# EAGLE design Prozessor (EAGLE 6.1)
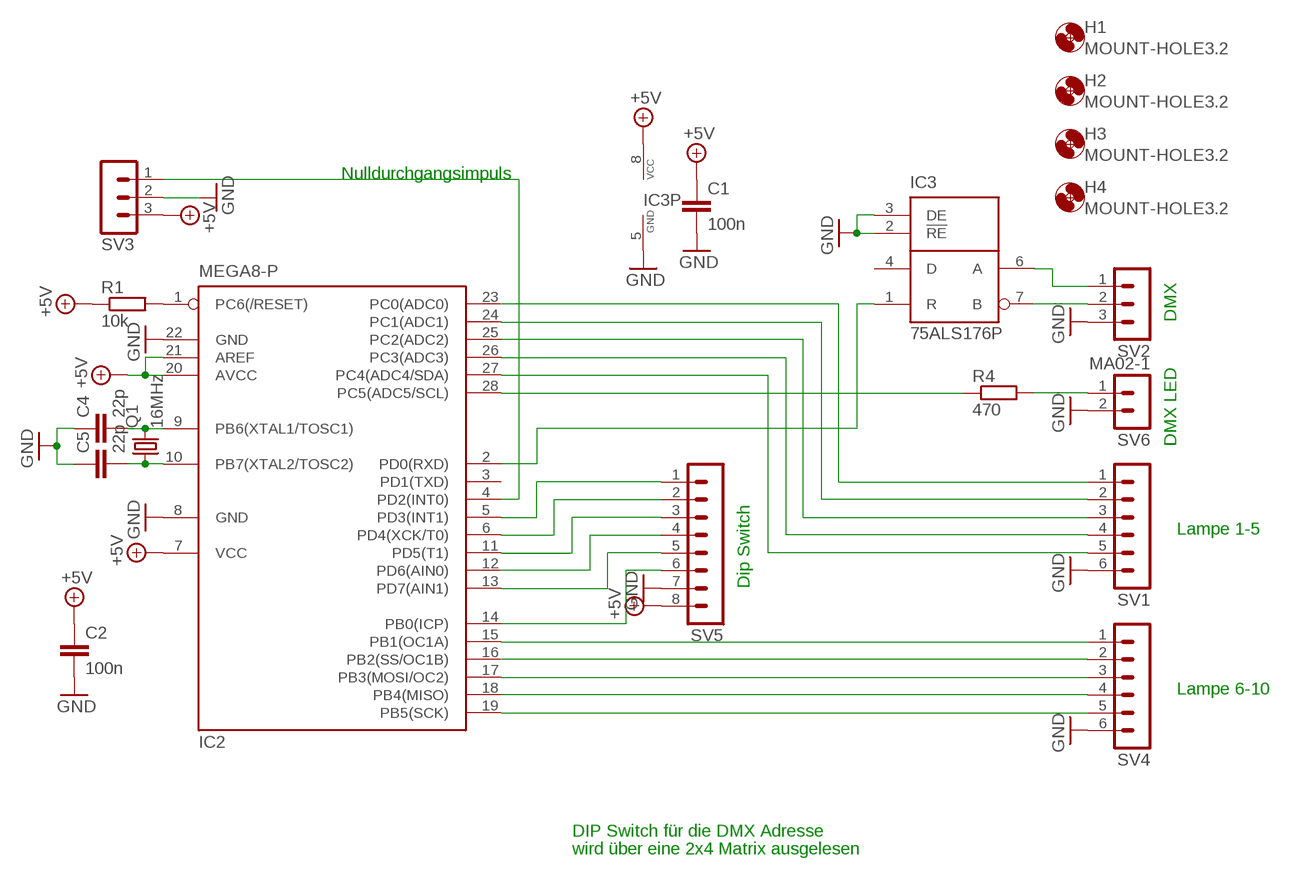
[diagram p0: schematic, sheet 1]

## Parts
C1  100n  C-EU050-025X075  [C050-025X075]
C2  100n  C-EU050-025X075  [C050-025X075]
C4  22p  C-EU025-025X050  [C025-025X050]
C5  22p  C-EU025-025X050  [C025-025X050]
H1  MOUNT-HOLE3.2  [3,2]
H2  MOUNT-HOLE3.2  [3,2]
H3  MOUNT-HOLE3.2  [3,2]
H4  MOUNT-HOLE3.2  [3,2]
IC2  MEGA8-P  [DIL28-3]
IC3  75ALS176P  [DIL08]
Q1  16MHz  CRYSTALHC49U70  [HC49U70]
R1  10k  R-EU_0204/7  [0204/7]
R4  470  R-EU_0204/7  [0204/7]
SV1  MA06-1  [MA06-1]
SV2  MA03-1  [MA03-1]
SV3  MA03-1  [MA03-1]
SV4  MA06-1  [MA06-1]
SV5  MA08-1  [MA08-1]
SV6  MA02-1  [MA02-1]

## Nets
+5V: C1.1 C2.1 IC2.7(VCC) IC2.20(AVCC) IC2.21(AREF) IC3.8(VCC) R1.1 SV3.3 SV5.8
GND: C1.2 C2.2 C4.1 C5.1 IC2.8(GND) IC2.22(GND) IC3.2(!RE) IC3.3(DE) IC3.5(GND) SV1.6 SV2.3 SV3.2 SV4.6 SV5.7 SV6.2
N$1: IC2.12(PD6(AIN0)) SV5.4
N$2: IC2.13(PD7(AIN1)) SV5.5
N$3: IC2.11(PD5(T1)) SV5.3
N$4: IC2.6(PD4(XCK/T0)) SV5.2
N$5: IC2.5(PD3(INT1)) SV5.1
N$6: IC2.27(PC4(ADC4/SDA)) SV1.5
N$7: IC2.23(PC0(ADC0)) SV1.1
N$8: IC2.4(PD2(INT0)) SV3.1
N$9: R4.2 SV6.1
N$10: C4.2 IC2.9(PB6(XTAL1/TOSC1)) Q1.2
N$11: C5.2 IC2.10(PB7(XTAL2/TOSC2)) Q1.1
N$12: IC2.14(PB0(ICP)) SV5.6
N$13: IC2.19(PB5(SCK)) SV4.5
N$14: IC2.18(PB4(MISO)) SV4.4
N$15: IC2.17(PB3(MOSI/OC2)) SV4.3
N$16: IC2.16(PB2(SS/OC1B)) SV4.2
N$17: IC2.15(PB1(OC1A)) SV4.1
N$18: IC2.1(PC6(/RESET)) R1.2
N$19: IC2.24(PC1(ADC1)) SV1.2
N$20: IC2.25(PC2(ADC2)) SV1.3
N$21: IC2.26(PC3(ADC3)) SV1.4
N$23: IC2.2(PD0(RXD)) IC3.1(R)
N$24: IC3.6(A) SV2.1
N$25: IC3.7(B) SV2.2
N$27: IC2.28(PC5(ADC5/SCL)) R4.1
Unconnected: IC2.3(PD1(TXD)) IC3.4(D)

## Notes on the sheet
- Nulldurchgangsimpuls
- DMX
- DMX LED
- Lampe 1-5
- Dip Switch
- Lampe 6-10
- DIP Switch für die DMX Adresse
- wird über eine 2x4 Matrix ausgelesen

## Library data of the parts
C1 C2 = rcl:C-EU: CAPACITOR, European symbol
C4 C5 = resistor:C-EU: CAPACITOR, European symbol
H1-H4 = holes:MOUNT-HOLE: MOUNTING HOLE with drill center marker
IC2 = atmel:MEGA8-P: MICROCONTROLLER 8 Kbytes FLASH, 1 kbytes SRAM, 512 bytes EEPROM, USART, 4-channel 10 bit ADC, 2-channel 8 bit ADC Pin compatible with Atmega48, ATMega88, ATMega168 Source: avr.lbr
IC3 = texas:75ALS176: DIFFERENTIAL BUS TRANSCEIVERS TIA/EIA-422-B, TIA/EIA-422-B + TIA/EIA-422-B TIA/EIA-422-B Operate at Data Rates up to 35 Mbaud Source: http://focus.ti.com/lit/ds/symlink/sn65als176.pdf
Q1 = crystal:CRYSTAL: CRYSTAL
R1 R4 = resistor:R-EU_: RESISTOR, European symbol
SV1 SV4 = con-lstb:MA06-1: PIN HEADER; OC_FARNELL: unknown; OC_NEWARK: unknown
SV2 SV3 = con-lstb:MA03-1: PIN HEADER; OC_FARNELL: unknown; OC_NEWARK: unknown
SV5 = con-lstb:MA08-1: PIN HEADER; OC_FARNELL: unknown; OC_NEWARK: unknown
SV6 = con-lstb:MA02-1: PIN HEADER

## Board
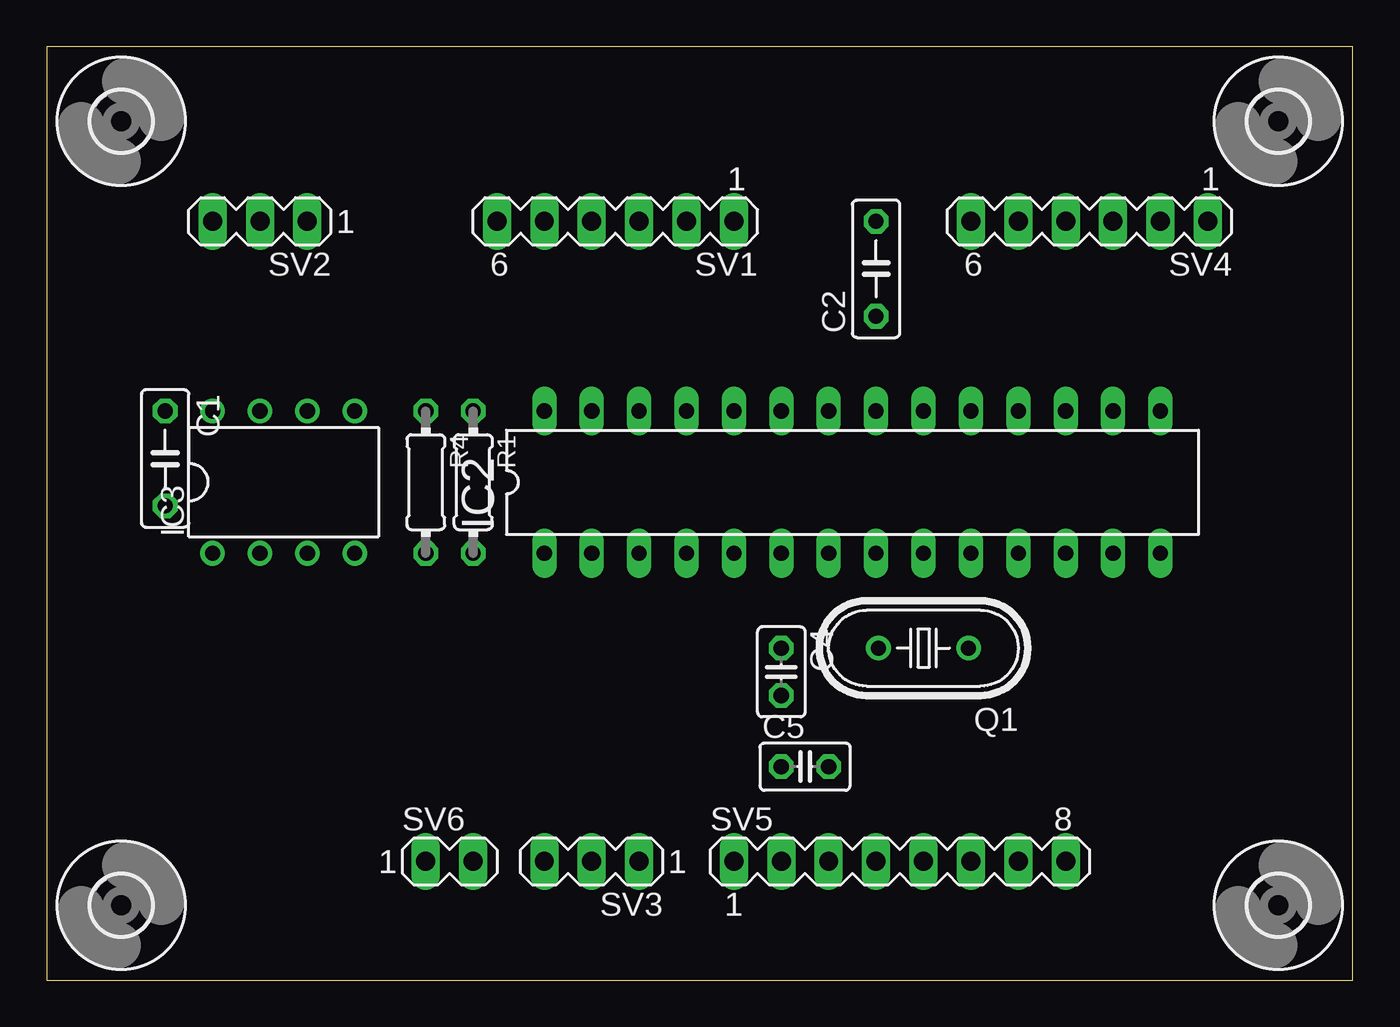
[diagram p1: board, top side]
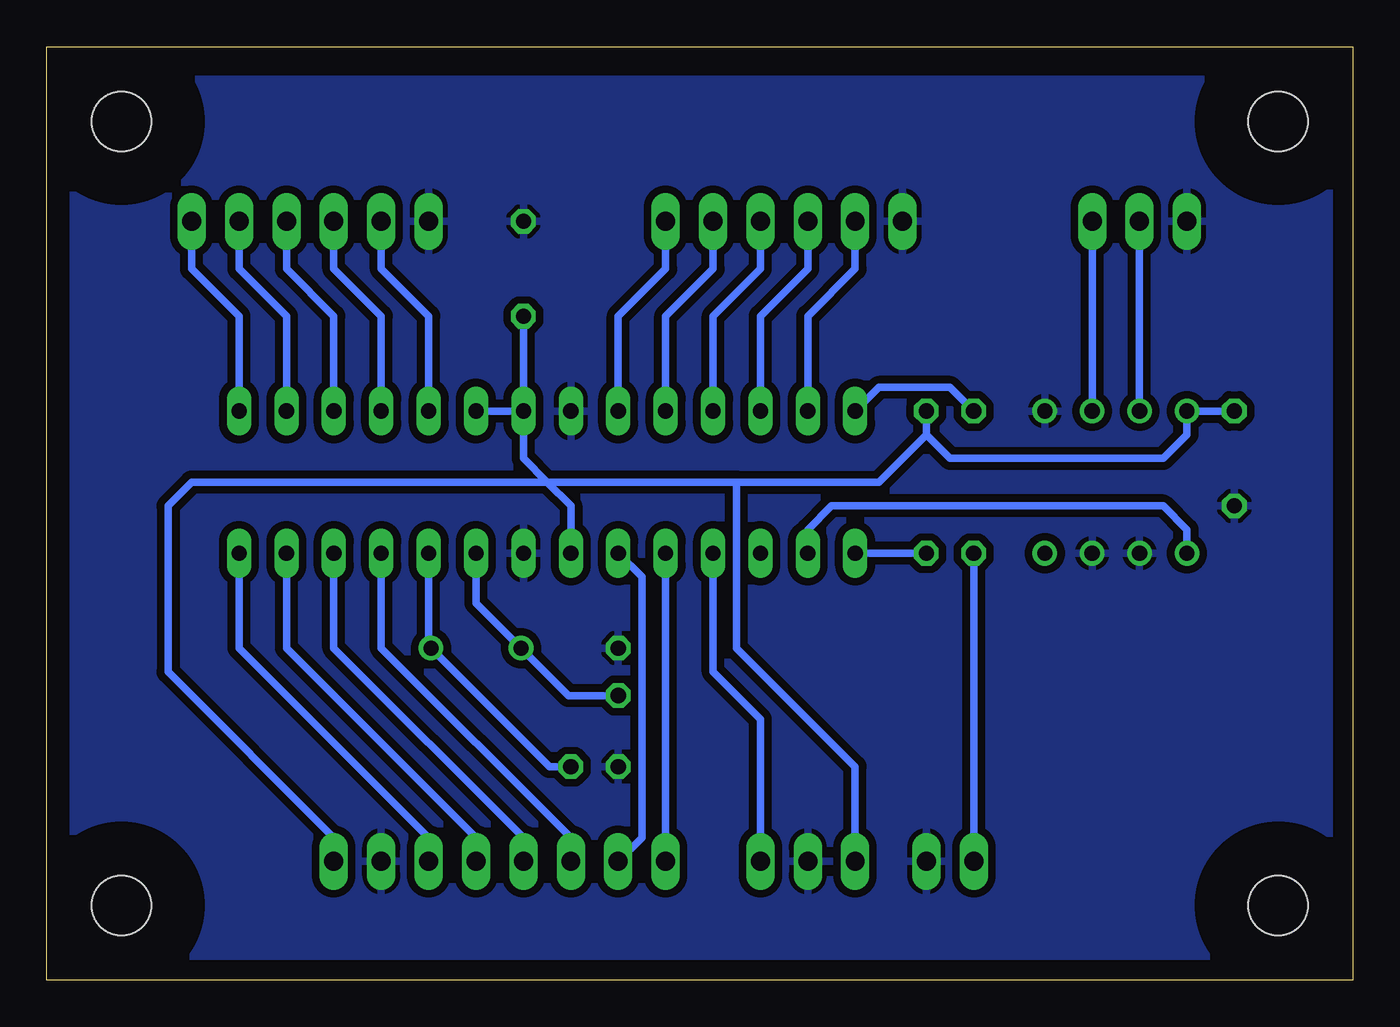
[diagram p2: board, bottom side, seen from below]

Size 70 x 50 mm. Coordinates in mm from the lower left corner, seen from the top.
Outline: 0,0 70,0 70,50 0,50 0,0
Copper layers (1*16): Top 0.035mm / dielectric 1.5mm / Bottom 0.035mm
Design rules: minimum track width 10mil, minimum drill 24mil, track to track 8mil, track to pad 8mil, pad to pad 8mil, via to via 8mil, smd to smd 8mil, copper to edge 40mil, drill to drill 8mil, minimum pad ring 10mil, minimum via ring 8mil, stop-mask expansion 4mil, vias tented up to drill 0mil, thermal gap 10mil

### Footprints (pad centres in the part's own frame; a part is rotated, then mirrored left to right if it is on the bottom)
C050-025X075 = drill 0.813 octagon: 1 -2.54,0; 2 2.54,0
C025-025X050 = drill 0.813 octagon: 1 -1.27,0; 2 1.27,0
3,2 = hole 3.2: 0,0
DIL28-3 = drill 0.813 long: 1 -16.51,-3.81; 2 -13.97,-3.81; 3 -11.43,-3.81; 4 -8.89,-3.81; 5 -6.35,-3.81; 6 -3.81,-3.81; 7 -1.27,-3.81; 8 1.27,-3.81; 9 3.81,-3.81; 10 6.35,-3.81; 11 8.89,-3.81; 12 11.43,-3.81; 13 13.97,-3.81; 14 16.51,-3.81; 15 16.51,3.81; 16 13.97,3.81; 17 11.43,3.81; 18 8.89,3.81; 19 6.35,3.81; 20 3.81,3.81; 21 1.27,3.81; 22 -1.27,3.81; 23 -3.81,3.81; 24 -6.35,3.81; 25 -8.89,3.81; 26 -11.43,3.81; 27 -13.97,3.81; 28 -16.51,3.81
DIL08 = drill 0.813 pad 1.27: 1 -3.81,-3.81; 2 -1.27,-3.81; 3 1.27,-3.81; 4 3.81,-3.81; 5 3.81,3.81; 6 1.27,3.81; 7 -1.27,3.81; 8 -3.81,3.81
HC49U70 = drill 0.813: 1 -2.413,0; 2 2.413,0
0204/7 = drill 0.813 octagon: 1 -3.81,0; 2 3.81,0
MA06-1 = drill 1.016 long: 1 -6.35,0; 2 -3.81,0; 3 -1.27,0; 4 1.27,0; 5 3.81,0; 6 6.35,0
MA03-1 = drill 1.016 long: 1 -2.54,0; 2 0,0; 3 2.54,0
MA08-1 = drill 1.016 long: 1 -8.89,0; 2 -6.35,0; 3 -3.81,0; 4 -1.27,0; 5 1.27,0; 6 3.81,0; 7 6.35,0; 8 8.89,0
MA02-1 = drill 1.016 long: 1 -1.27,0; 2 1.27,0

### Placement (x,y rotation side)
C1  6.35,27.94 270 top
C2  44.45,38.1 90 top
C4  39.37,16.51 270 top
C5  40.64,11.43 0 top
H1  4,4 0 top
H2  4,46 0 top
H3  66,4 0 top
H4  66,46 0 top
IC2  43.18,26.67 0 top
IC3  12.7,26.67 0 top
Q1  46.99,17.78 180 top
R1  22.86,26.67 270 top
R4  20.32,26.67 270 top
SV1  30.48,40.64 180 top
SV2  11.43,40.64 180 top
SV3  29.21,6.35 180 top
SV4  55.88,40.64 180 top
SV5  45.72,6.35 0 top
SV6  21.59,6.35 0 top

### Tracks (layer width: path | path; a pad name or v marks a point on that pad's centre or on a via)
+5V
  Bottom 0.406: IC2.21 IC2.20 | IC2.7 41.91,25.4 43.18,26.67 | 43.18,26.67 44.45,27.94 IC2.21 | C1.1 IC3.8 8.89,29.21 10.16,27.94 21.59,27.94 22.86,29.21 | IC2.21 C2.1 | 33.02,26.67 43.18,26.67 | SV3.3 26.67,11.43 33.02,17.78 33.02,26.67 | 22.86,29.21 R1.1 | 33.02,26.67 25.4,26.67 22.86,29.21 | 43.18,26.67 62.23,26.67 63.5,25.4 63.5,16.51 54.61,7.62 SV5.8
GND
  pour Bottom (isolate 0.406): 1.27,1.27 1.27,48.26 68.58,48.26 68.58,41.91 68.58,1.27
N$1
  Bottom 0.406: SV5.4 44.45,7.62 54.61,17.78 IC2.12
N$2
  Bottom 0.406: SV5.5 46.99,7.62 57.15,17.78 IC2.13
N$3
  Bottom 0.406: SV5.3 41.91,7.62 52.07,17.78 IC2.11
N$4
  Bottom 0.406: IC2.6 38.1,21.59 38.1,7.62 SV5.2
N$5
  Bottom 0.406: SV5.1 IC2.5
N$6
  Bottom 0.406: SV1.5 26.67,38.1 29.21,35.56 IC2.27
N$7
  Bottom 0.406: SV1.1 36.83,38.1 39.37,35.56 IC2.23
N$8
  Bottom 0.406: SV3.1 31.75,13.97 34.29,16.51 IC2.4
N$9
  Bottom 0.406: SV6.1 R4.2
N$10
  Bottom 0.406: C4.2 42.04,15.24 Q1.2 46.99,20.19 IC2.9
N$11
  Bottom 0.406: C5.2 43.05,11.43 Q1.1 49.53,17.91 IC2.10
N$12
  Bottom 0.406: SV5.6 49.53,7.62 59.69,17.78 IC2.14
N$13
  Bottom 0.406: SV4.5 52.07,38.1 49.53,35.56 IC2.19
N$14
  Bottom 0.406: SV4.4 54.61,38.1 52.07,35.56 IC2.18
N$15
  Bottom 0.406: SV4.3 57.15,38.1 54.61,35.56 IC2.17
N$16
  Bottom 0.406: SV4.2 59.69,38.1 57.15,35.56 IC2.16
N$17
  Bottom 0.406: SV4.1 62.23,38.1 59.69,35.56 IC2.15
N$18
  Bottom 0.406: R1.2 IC2.1
N$19
  Bottom 0.406: SV1.2 34.29,38.1 36.83,35.56 IC2.24
N$20
  Bottom 0.406: SV1.3 31.75,38.1 34.29,35.56 IC2.25
N$21
  Bottom 0.406: SV1.4 29.21,38.1 31.75,35.56 IC2.26
N$23
  Bottom 0.406: IC2.2 29.21,24.13 27.94,25.4 10.16,25.4 8.89,24.13 IC3.1
N$24
  Bottom 0.406: IC3.6 SV2.1
N$25
  Bottom 0.406: IC3.7 SV2.2
N$27
  Bottom 0.406: R4.1 21.59,31.75 25.4,31.75 IC2.28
